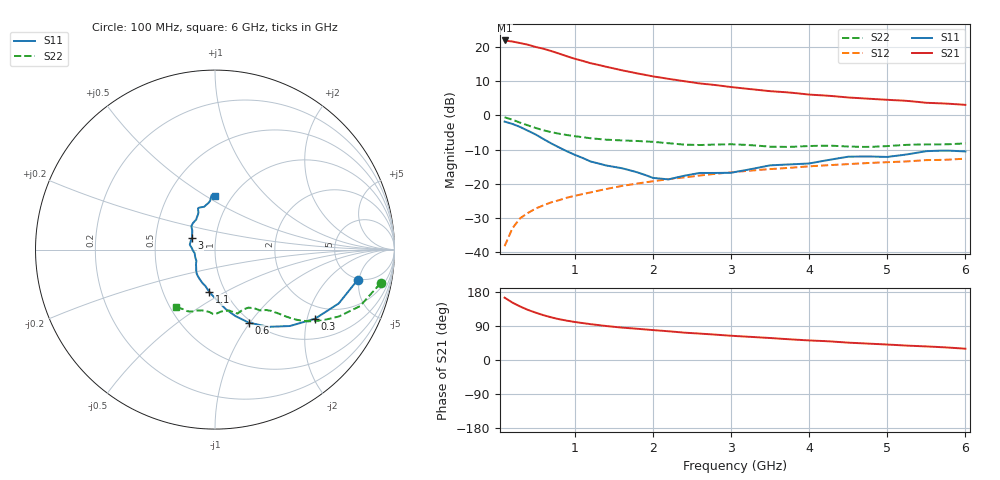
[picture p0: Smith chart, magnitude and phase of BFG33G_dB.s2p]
! Created Sun Mar 29 23:17:58 2009
# hz S db R 50
! 2 Port Network Data from SP1.SP block
! freq  dbS11  angS11  dbS21  angS21  dbS12  angS12  dbS22  angS22
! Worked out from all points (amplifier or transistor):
!   60 points, 100 MHz to 6 GHz, reference 50 ohm
!   highest |S21| = 22.1 dB at 100 MHz (marker M1)
!   |S21| within 3 dB of that: start of sweep to 680.1 MHz
!   unconditionally stable (mu >= 1): 1.147 GHz to end of sweep
!   at 1.1 GHz: K = 0.98, MSG = 19.6 dB, |S12| = -23.1 dB
!   at 3.1 GHz: K = 1.25, MAG = 9.3 dB, |S12| = -16.5 dB
!   at 6 GHz: K = 1.36, MAG = 4.3 dB, |S12| = -12.7 dB
!   lowest NFmin = 3.10 dB at 100 MHz
!   S11 on the Smith chart (normalised r, x): 100 MHz: 4.85, -4.80; 300 MHz: 1.57, -2.23; 600 MHz: 0.97, -0.99; 1.1 GHz: 0.84, -0.42; 3 GHz: 0.77, +0.10; 6 GHz: 0.84, +0.55
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1e8  -1.80 -11.9  22.06 164.5  -38.42 79.3  -0.53 -11.5
2e8  -2.48 -23.5  21.74 151.5  -33.15 72.0  -1.24 -21.3
3e8  -3.39 -34.7  21.29 141.1  -30.17 67.2  -2.11 -28.4
4e8  -4.50 -45.6  20.79 132.1  -28.64 63.8  -2.93 -33.6
5e8  -5.61 -55.2  20.13 124.8  -27.33 61.8  -3.69 -37.7
6e8  -6.96 -65.1  19.61 118.1  -26.38 61.1  -4.36 -40.4
7e8  -8.25 -73.0  18.92 112.4  -25.51 60.5  -4.91 -42.2
8e8  -9.42 -79.6  18.18 107.6  -24.88 60.4  -5.37 -43.5
9e8  -10.54 -85.3  17.39 103.7  -24.15 60.3  -5.75 -44.5
1e9  -11.57 -91.3  16.67 100.3  -23.61 60.3  -6.09 -45.5
1.1e9  -12.49 -97.8  16.05 97.5  -23.10 60.2  -6.38 -46.5
1.2e9  -13.51 -104.4  15.38 94.6  -22.62 60.2  -6.69 -47.5
1.3e9  -14.09 -111.3  14.87 92.2  -22.10 60.1  -6.90 -48.6
1.5e9  -15.09 -122.8  13.83 87.6  -21.16 60.0  -7.22 -50.9
1.8e9  -16.71 -135.9  12.36 82.4  -20.00 59.9  -7.49 -53.4
2.1e9  -18.56 -159.4  11.14 77.3  -19.02 59.0  -7.95 -55.5
2.6e9  -16.89 168.9  9.41 69.7  -17.65 57.1  -8.68 -64.9
3e9  -16.83 153.0  8.36 64.0  -16.71 55.5  -8.45 -70.6
3.1e9  -16.41 148.0  8.12 62.8  -16.50 55.2  -8.55 -71.4
4.1e9  -13.68 119.0  6.01 50.7  -14.81 51.2  -8.92 -89.5
5.1e9  -11.89 101.0  4.49 39.7  -13.64 46.9  -8.84 -108.7
6e9  -10.57 89.6  3.13 29.8  -12.69 42.9  -8.20 -124.4
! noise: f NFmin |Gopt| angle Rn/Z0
1e+08  3.1  0.528  5.3  1.18
7e+08  3.1  0.5076  8.26  1.24
1.4e+09  3.3  0.4534  23.26  1.19
2e+09  3.6  0.418  39.1  0.98
2.7e+09  3.6  0.418  39.1  0.98
3.3e+09  3.6  0.418  39.1  0.98
4e+09  3.6  0.418  39.1  0.98
4.6e+09  3.6  0.418  39.1  0.98
5.3e+09  3.6  0.418  39.1  0.98
6e+09  3.6  0.418  39.1  0.98
